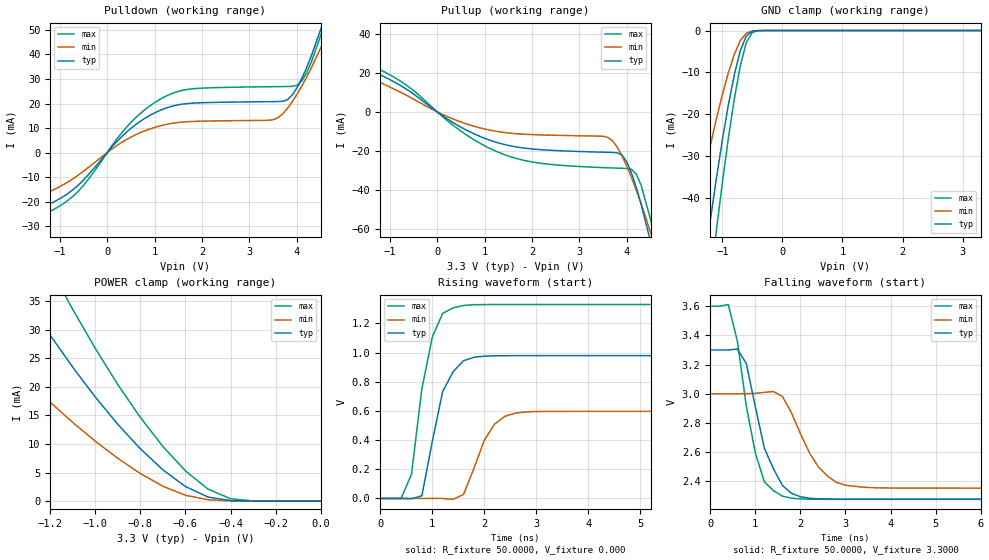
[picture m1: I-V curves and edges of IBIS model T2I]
| IBIS file t2i.ibs created by s2ibis2 version 1.1
| North Carolina State University Electronics Research Laboratory  1995
[IBIS ver]   2.1
[File name]   t2i.ibs
[File Rev]   1.0
[Date]   Wednesday, March 29, 2000
[Source]   From silicon level SPICE at TOSHIBA.
[Notes]   This model does not include the values of Package Model
[Disclaimer]   None.
[Copyright]   Copyright(C) TOSHIBA Corp. 1996-2000. All Rights Reserved
|   Component TC260C
[Component]   TC260C
[Manufacturer]   TOSHIBA
[Package]
| variable   typ   min   max
R_pkg   1.0000f   NA   NA
L_pkg   1.0000fH   NA   NA
C_pkg   1.0000fF   NA   NA
[Pin]  signal_name   model_name   R_pin   L_pin   C_pin
Z   Z   T2I
VDDS   VDDS   POWER
VSS   VSS   GND
| Models and submodels in the file (1): T2I (3-state)
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|   Model T2I
[Model]   T2I
Model_type   3-state
Polarity   Non-Inverting
C_comp   4.2000pF   NA   NA
Vmeas = 1.40V
|Variable   typ   min   max
[Voltage range]  3.3   3.0   3.6
[Temperature Range]   25.0000   100.0000   0.000
[Pullup Reference]   3.3000V   3.0000V   3.6000V
[Pulldown Reference]   0.000V   0.000V   0.000V
[POWER Clamp Reference]   3.3000V   3.0000V   3.6000V
[GND Clamp Reference]   0.000V   0.000V   0.000V
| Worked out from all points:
|   slope of the pulldown table from 0 to 0.495 V, typ, clamps not added: 50.5 ohm
|   slope of the pullup table from 0 to 0.495 V, typ, clamps not added: 63.9 ohm
|   GND clamp passes 1 mA (typ) near -0.57 V on its own axis
|   POWER clamp passes 1 mA (typ) near -0.52 V on its own axis
|   rising waveform, R_fixture 50.0000, V_fixture 0.000: 20-80 % time 378ps typ, 437ps min, 342ps max; typ from 0 V to 0.978 V
|   falling waveform, R_fixture 50.0000, V_fixture 3.3000: 20-80 % time 534ps typ, 652ps min, 440ps max; typ from 3.3 V to 2.28 V
[Pulldown]
| voltage   I(typ)   I(min)   I(max)
-3.3V     -29.37mA   -29.01mA   -32.31mA
-1.9V     -25.53mA   -21.44mA   -28.71mA
-1V       -18.77mA   -13.85mA   -21.76mA
-500mV    -11.12mA   -7.595mA   -13.35mA
500mV     9.878mA    6.294mA    12.28mA
1.3V      18.52mA    11.69mA    23.54mA
3.5V      20.78mA    13.39mA    26.86mA
3.8V      21.56mA    18.01mA    26.94mA
4.1V      30.06mA    26.99mA    29.13mA
4.5V      50.11mA    42.6mA     47.62mA
4.7V      62.45mA    51.64mA    60.99mA
6.6V      227.2mA    181.8mA    250.9mA
[Pullup]
| voltage   I(typ)   I(min)   I(max)
-3.3V     35.88mA    43.25mA    36.87mA
-2.1V     27.55mA    25.61mA    29.91mA
-1.1V     17.77mA    13.9mA     20.3mA
600mV     -9.13mA    -6.021mA   -11.53mA
1.8V      -18.45mA   -11.4mA    -24.67mA
3.6V      -20.71mA   -13.11mA   -28.63mA
3.9V      -22.18mA   -22.69mA   -28.89mA
4.2V      -38.9mA    -40.21mA   -31.94mA
4.3V      -47.34mA   -47.03mA   -37.57mA
4.5V      -66.59mA   -61.78mA   -55.16mA
4.7V      -88.01mA   -77.77mA   -77.42mA
6.6V      -315mA     -263.4mA   -330mA
[GND_clamp]
| voltage   I(typ)   I(min)   I(max)
-3.3V     -292.8mA   -217.8mA   -337.5mA
-1.5V     -77.97mA   -49.07mA   -98.95mA
-1.3V     -55.88mA   -34.36mA   -72.74mA
-1.2V     -45.43mA   -27.57mA   -60.12mA
-1.1V     -35.51mA   -21.22mA   -47.98mA
-900mV    -17.87mA   -10.14mA   -25.85mA
-800mV    -10.56mA   -5.698mA   -16.34mA
-700mV    -4.792mA   -2.412mA   -8.394mA
-600mV    -1.302mA   -649uA     -2.833mA
-500mV    -170.7uA   -108.2uA   -443.3uA
-400mV    -13.58uA   -13.64uA   -33.16uA
3.3V      153.8pA    4.347uA    -1.02nA
[POWER_clamp]
| voltage   I(typ)   I(min)   I(max)
-3.3V     184.7mA    132.7mA    223.8mA
-1.7V     61.09mA    38.14mA    81.03mA
-1.6V     54.23mA    33.59mA    72.55mA
-1.3V     34.91mA    21.05mA    48.28mA
-1.2V     28.99mA    17.28mA    40.71mA
-1.1V     23.4mA     13.75mA    33.49mA
-900mV    13.42mA    7.478mA    20.36mA
-800mV    9.146mA    4.821mA    14.61mA
-600mV    2.551mA    1.023mA    5.293mA
-500mV    720.3uA    246uA      2.105mA
-400mV    92.66uA    36.99uA    415.4uA
0V        153.8pA    711.8pA    166.4pA
[Ramp]
| variable   typ   min   max
dV/dt_r   0.5871/0.3313n   0.3581/0.4089n   0.7975/0.3069n
dV/dt_f   0.6138/0.4767n   0.3881/0.6394n   0.7941/0.4120n
R_load = 50.0000
[Rising Waveform]
R_fixture = 50.0000
V_fixture = 0.000
V_fixture_min = 0.000
V_fixture_max = 0.000
| time   V(typ)   V(min)   V(max)
0s        0V         0V         0V
400ps     25.65uV    -34.07uV   -32.64uV
600ps     -2.657mV   19.97uV    165.3mV
800ps     18.2mV     107.4uV    751.5mV
1ns       389.6mV    285.4uV    1.105V
1.2ns     732.7mV    -392.7uV   1.268V
1.4ns     868.1mV    -6.149mV   1.306V
2.2ns     977.4mV    510mV      1.329V
2.6ns     978.4mV    584.5mV    1.329V
10ns      978.5mV    596.8mV    1.329V
[Falling Waveform]
R_fixture = 50.0000
V_fixture = 3.3000
V_fixture_min = 3.0000
V_fixture_max = 3.6000
| time   V(typ)   V(min)   V(max)
0s        3.3V       3V         3.6V
400ps     3.3V       3V         3.612V
600ps     3.307V     3V         3.364V
800ps     3.207V     3.001V     2.916V
1ns       2.911V     3.003V     2.594V
1.2ns     2.627V     3.01V      2.396V
1.6ns     2.372V     2.982V     2.299V
2.4ns     2.28V      2.499V     2.277V
3ns       2.277V     2.373V     2.276V
10ns      2.277V     2.353V     2.276V
